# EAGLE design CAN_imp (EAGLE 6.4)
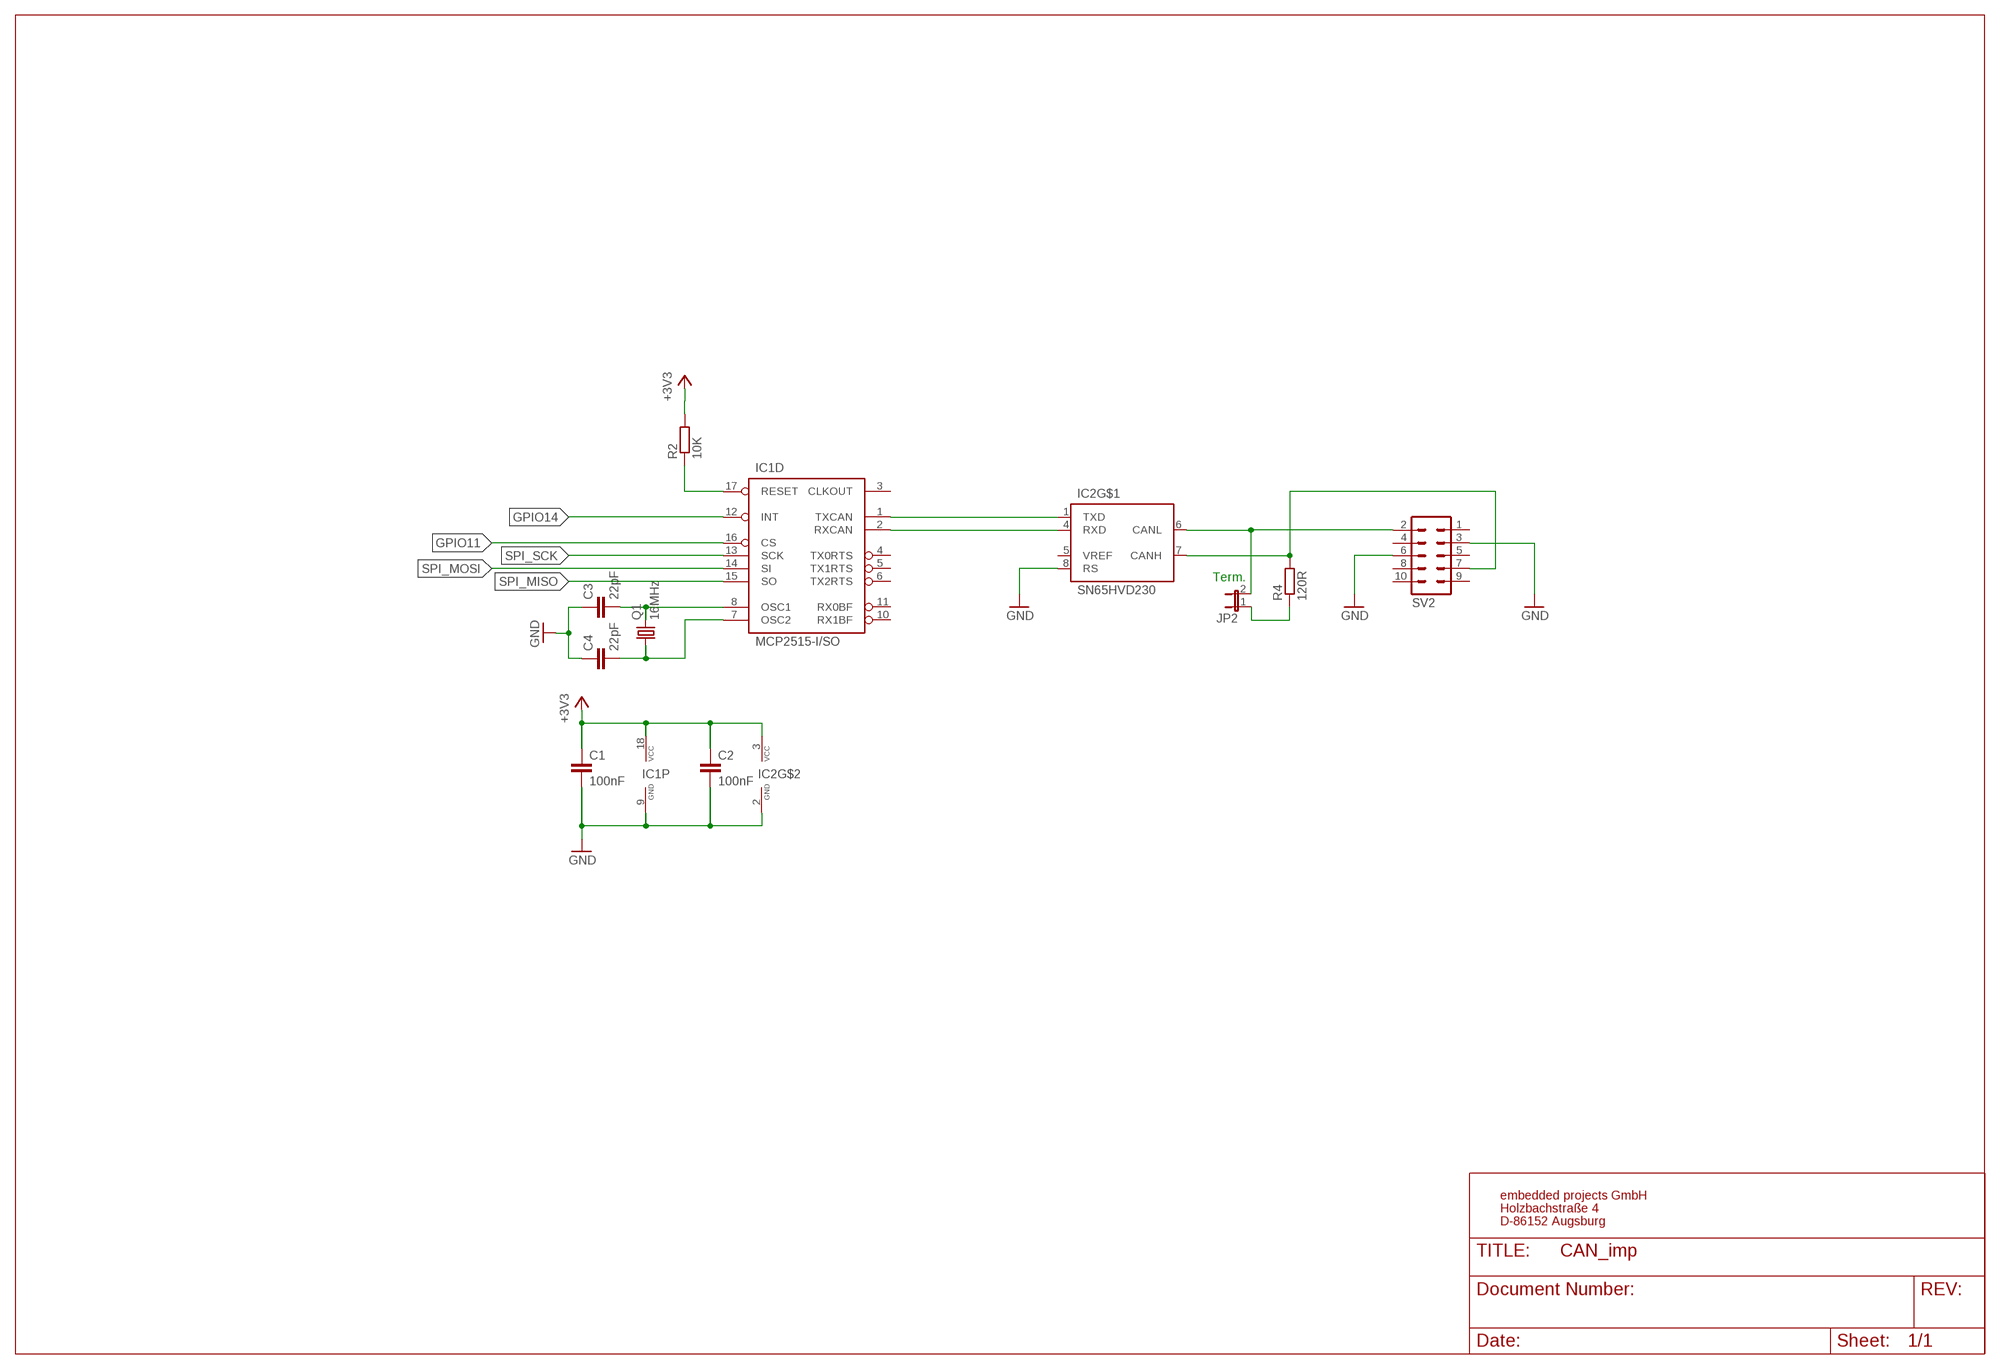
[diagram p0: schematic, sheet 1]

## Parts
C1  100nF  C-EUC0805  [C0805]
C2  100nF  C-EUC0805  [C0805]
C3  22pF  C-EUC0805  [C0805]
C4  22pF  C-EUC0805  [C0805]
IC1  MCP2515-I/SO  MCP2515SO  [SO-18W]
IC2  SN65HVD230  MCP2551SO8  [SO08]
JP2  JP1E  [JP1]
Q1  16MHz  CRYSTALHC49UP  [HC49UP]
R2  10K  R-EU_R0805  [R0805]
R4  120R  R-EU_R0805  [R0805]
SV2  ML10  [ML10]

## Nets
+3V3: C1.1 C2.1 IC1.18(P:VCC) IC2.3(VCC) R2.2
CANH: IC2.7(CANH) R4.2 SV2.7
CANL: IC2.6(CANL) JP2.2 SV2.2
GND: C1.2 C2.2 C3.1 C4.1 IC1.9(P:GND) IC2.2(GND) IC2.8(RS) SV2.3 SV2.6
GPIO11: IC1.16(D:CS)
GPIO14: IC1.12(D:INT)
N$2: C3.2 IC1.8(D:OSC1) Q1.2
N$3: C4.2 IC1.7(D:OSC2) Q1.1
N$4: IC1.1(D:TXCAN) IC2.1(TXD)
N$5: IC1.2(D:RXCAN) IC2.4(RXD)
N$6: IC1.17(D:RESET) R2.1
N$11: JP2.1 R4.1
SPI_MISO: IC1.15(D:SO)
SPI_MOSI: IC1.14(D:SI)
SPI_SCK: IC1.13(D:SCK)
Unconnected: IC1.3(D:CLKOUT) IC1.4(D:TX0RTS) IC1.5(D:TX1RTS) IC1.6(D:TX2RTS) IC1.10(D:RX1BF) IC1.11(D:RX0BF) IC2.5(VREF) SV2.1 SV2.4 SV2.5 SV2.8 SV2.9 SV2.10

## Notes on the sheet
- Term.
- embedded projects GmbH
- Holzbachstraße 4
- D-86152 Augsburg

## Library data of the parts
C1-C4 = rcl:C-EU: CAPACITOR, European symbol
IC1 = can:MCP2515: MC2515 Stand-Alone CAN Controller With SPI Interface, Microchip; FARNELL: 1292239
IC2 = can:MCP2551: CAN Tranceiver Microchip; FARNELL: 1103105
JP2 = jumper:JP1E: JUMPER
Q1 = crystal:CRYSTAL: CRYSTAL; OC_FARNELL: unknown; OC_NEWARK: unknown
R2 R4 = rcl:R-EU_: RESISTOR, European symbol
SV2 = con-ml:ML10: HARTING

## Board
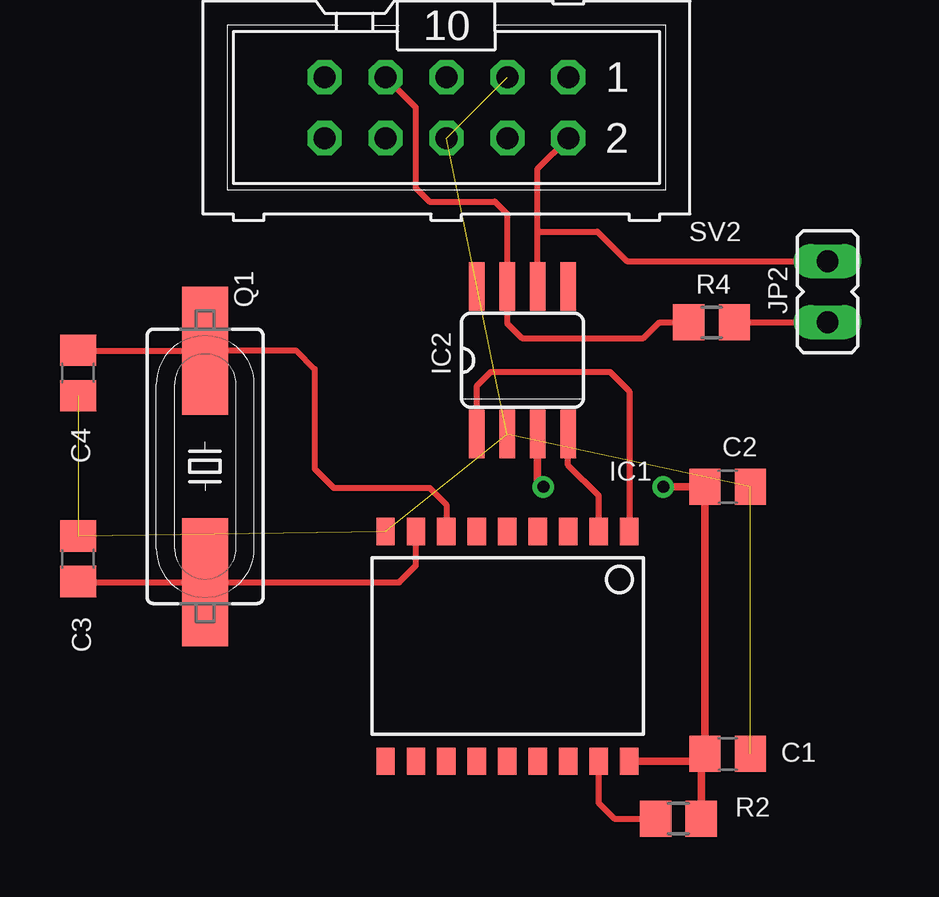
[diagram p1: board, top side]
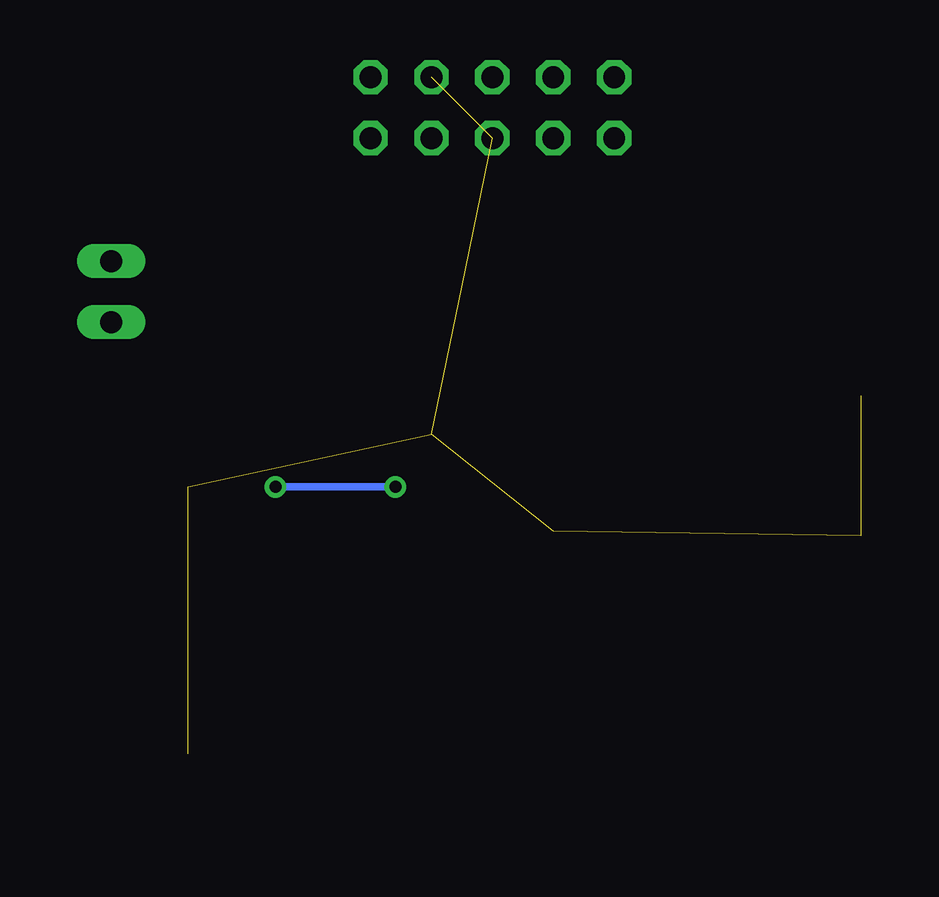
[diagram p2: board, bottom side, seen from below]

No outline drawn. Coordinates in mm, seen from the top.
Copper layers (1*16): Top 0.035mm / dielectric 1.5mm / Bottom 0.035mm
Design rules "default *": minimum track width 10mil, minimum drill 24mil, track to track 8mil, track to pad 8mil, pad to pad 8mil, via to via 8mil, smd to smd 8mil, copper to edge 20mil, drill to drill 8mil, minimum pad ring 10mil, minimum via ring 8mil, stop-mask expansion 2mil, vias tented up to drill 40mil, thermal gap 10mil

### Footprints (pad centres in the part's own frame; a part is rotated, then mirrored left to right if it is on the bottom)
C0805 = smd 1.3 x 1.5: 1 -0.95,0; 2 0.95,0
SO-18W = smd 0.762 x 1.143: 1 -5.08,-4.788; 2 -3.81,-4.788; 3 -2.54,-4.788; 4 -1.27,-4.788; 5 0,-4.788; 6 1.27,-4.788; 7 2.54,-4.788; 8 3.81,-4.788; 9 5.08,-4.788; 10 5.08,4.788; 11 3.81,4.788; 12 2.54,4.788; 13 1.27,4.788; 14 0,4.788; 15 -1.27,4.788; 16 -2.54,4.788; 17 -3.81,4.788; 18 -5.08,4.788
SO08 = smd 0.66 x 2.032: 1 -1.905,-3.073; 2 -0.635,-3.073; 3 0.635,-3.073; 4 1.905,-3.073; 5 1.905,3.073; 6 0.635,3.073; 7 -0.635,3.073; 8 -1.905,3.073
JP1 = drill 0.914 long: 1 0,-1.27; 2 0,1.27
HC49UP = smd 5.334 x 1.93: 1 -4.826,0; 2 4.826,0
R0805 = smd 1.3 x 1.5: 1 -0.95,0; 2 0.95,0
ML10 = drill 0.914 octagon: 1 -5.08,-1.27; 2 -5.08,1.27; 3 -2.54,-1.27; 4 -2.54,1.27; 5 0,-1.27; 6 0,1.27; 7 2.54,-1.27; 8 2.54,1.27; 9 5.08,-1.27; 10 5.08,1.27

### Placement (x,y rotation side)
C1  30.72,13.67 0 top
C2  30.72,24.8 0 top
C3  3.64,21.8 270 top
C4  3.64,29.54 90 top
IC1  21.54,18.15 180 top
IC2  22.17,30.07 0 top
JP2  34.89,32.93 0 top
Q1  8.94,25.65 270 top
R2  28.67,10.97 0 top
R4  30.05,31.65 180 top
SV2  19,40.6 180 top

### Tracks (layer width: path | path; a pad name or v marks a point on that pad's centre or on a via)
+3V3  (via drill 0.5)
  Top 0.305: R2.2 29.62,13.52 C1.1 | IC1.18 27.92,13.36 29.46,13.36 C1.1 | C1.1 29.77,16.13 | 29.77,16.13 29.77,16.27 | 29.77,16.27 C2.1 v28.04,24.79 | IC2.3 22.8,25.02 v23.04,24.79 | 29.77,16.13 29.77,16.27
  Bottom 0.305: v28.04,24.79 v23.04,24.79
CANH
  Top 0.254: R4.2 27.88,31.65 27.22,30.99 22.16,30.99 21.54,31.61 IC2.7 21.54,36.16 21.02,36.68 18.29,36.68 17.73,37.24 17.73,40.6 SV2.7
CANL
  Top 0.254: IC2.6 22.8,35.35 | JP2.2 26.52,34.2 25.29,35.43 22.89,35.43 22.8,35.35 | 22.8,35.35 22.8,38.05 SV2.2
GND  (8 unrouted)
N$2
  Top 0.254: IC1.8 17.73,21.52 17.03,20.82 Q1.2 3.67,20.82 C3.2
N$3
  Top 0.254: C4.2 3.65,30.48 Q1.1 12.73,30.48 13.51,29.7 13.51,25.54 14.3,24.75 18.3,24.75 19,24.05 IC1.7
N$4
  Top 0.254: IC1.1 26.62,28.77 25.82,29.59 20.85,29.59 20.27,29 IC2.1
N$5
  Top 0.254: IC2.4 24.07,25.7 25.35,24.43 IC1.2
N$6
  Top 0.254: R2.1 26,10.97 25.35,11.62 IC1.17
N$11
  Top 0.254: R4.1 JP2.1

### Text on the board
tDocu: CANH | CANL | Term. | www.gnublin.org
